FUNCTION_BLOCK FB_SortingModule EXTENDS FB_Module
// Module to select via sensor, cylinder and axis
VAR_INPUT
		(* Variables to enable / disable diagnosis and temperature mode *)
	bCylinderDiag				: BOOL;
	bCylinderTemp				: BOOL;
	bCylinderRecord				: BOOL;
		(* Buttons *)
	bButtonCylToWorkIn			: BOOL;
	bButtonCylToBaseIn			: BOOL;
		(* Timer values *)
	tTimeOutCylinder			: TIME;
	tRecordIntervall			: TIME;
	tSensorDelay				: TIME;
	tMoveAxis					: TIME;					// Time to move axis
END_VAR
VAR_OUTPUT
	bToWork						: BOOL;
	bAtBase						: BOOL;
	bAtWork						: BOOL;
	bCylError					: BOOL;
	sCylErrorMsg				: STRING;
	aTemps						: ARRAY[1..100] OF LREAL;
	bSelected					: BOOL;
	bButtonCylToWorkOut			: BOOL;
	bButtonCylToBaseOut			: BOOL;
END_VAR
VAR
(* ================= Function block and interface instances ===================== *)
	
	fbSensorDelay				: FB_SignalHandlingDelay;
		(* Instances of cylinder function blocks *)
	fbCylinder					: FB_Cylinder;					// Without diagnosis and temperature mode
	fbCylinderDiag				: FB_CylinderDiag;				// With diagnosis of states
	fbCylinderTemp				: FB_CylinderTemp;				// With temperature mode
	fbCylinderTempDiag			: FB_CylinderTempDiag;			// With diagnosis of temperature
	fbCylinderTempRecord		: FB_CylinderTempRecord;		// With record of temperatures
		(* Interface instance of ICylinder for cylinder *)
	iCyl						: ICylinder;
	
		(***** Manual cylinder control *****)
	fbButtonCylToWork			: FB_SignalHandlingIntern;		// To move manually cylinder to work position
	fbButtonCylToBase			: FB_SignalHandlingIntern;		// To move manually cylinder to base position

(* ========================== COMMON VARIABLES =============================== *)
	fbTimerAxis					: TON;							// Timer to move axis in (SEMI-) AUTOMATIC mode	
	fbTriggerCylAtWork			: R_TRIG;						// To diagnose rising edge of being in work position
	eStateAuto					: E_StateSortingAuto;
END_VAR

// =========================================================
;
// =========================================================

METHOD PROTECTED M_ResetState
VAR_INPUT
END_VAR
// =========================================================

eStateAuto := eSortingAuto_DetectBox;

// =========================================================
END_METHOD

METHOD PUBLIC M_SetOutput
VAR_INPUT
END_VAR
// =========================================================
		// Calling method M_SetOutput of base class FB_Module via 'SUPER^.'
		
SUPER^.M_SetOutput();

// =========================================================
		// Sensor
		
fbSensorDelay.M_SetOutput();

// =========================================================
		// Cylinder buttons
		
fbButtonCylToWork.M_SetOutput();
fbButtonCylToBase.M_SetOutput();

// =========================================================
		// Output variables for cylinder
		
bToWork := iCyl.P_ToWork;			// Assigning global output variable to property of selected FB
									// Accessing property of selected FB via interface instance
bAtBase := iCyl.P_AtBasePos;
bAtWork := iCyl.P_AtWorkPos;

// =========================================================
		// Buttons
		
fbButtonCylToWork.bInput 	:= bButtonCylToWorkIn;
fbButtonCylToBase.bInput	:= bButtonCylToBaseIn;
bButtonCylToWorkOut 		:= fbButtonCylToWork.bOut;
bButtonCylToBaseOut 		:= fbButtonCylToBase.bOut;

// =========================================================
END_METHOD

METHOD PUBLIC M_Automatic
VAR_INPUT
END_VAR
// =========================================================
		// Selecting boxes via cylinder and axis

fbTimerAxis( PT := tMoveAxis );
fbTriggerCylAtWork( CLK := iCyl.P_AtWorkPos );			(***** Accessing property of FB via interface *****)

IF fbTriggerCylAtWork.Q THEN
	fbTimerAxis( IN := TRUE );
END_IF

IF bSelected THEN
	bSelected := FALSE;
END_IF

IF fbTimerAxis.Q THEN
	fbTimerAxis( IN := FALSE );
	
	bSelected 	:= TRUE;
	bHalt 		:= TRUE;
	
	M_Stop();
	
ELSIF fbTimerAxis.IN AND NOT bHalt THEN
	fbAxis.M_MoveFw();
END_IF

IF NOT bHaltDone THEN
	
	IF bHalt THEN
		M_Stop();
	END_IF
ELSE
	bHalt := FALSE;
	M_Stop();
END_IF

// =========================================================

CASE eStateAuto OF
	// =========================================================
	// Detecting a box
	eSortingAuto_DetectBox:	
	
			iCyl.M_MoveToBase();						(***** Calling method of FB via interface *****)
			
			IF fbSensorDelay.bOut THEN
				eStateAuto := eSortingAuto_CylToWork;
			END_IF
		
	// =========================================================
	// Moving cylinder to work position
	eSortingAuto_CylToWork:
	
			iCyl.M_MoveToWork();						(***** Calling method of FB via interface *****)
			
			IF iCyl.P_AtWorkPos THEN					(***** Accessing property of FB via interface *****)
				eStateAuto := eSortingAuto_CylToBase;
			END_IF
	
	// =========================================================
	// Moving cylinder back to base position
	eSortingAuto_CylToBase:
	
			iCyl.M_MoveToBase();						(***** Calling method of FB via interface *****)	
			
			IF iCyl.P_AtBasePos THEN					(***** Accessing property of FB via interface *****)
				eStateAuto := eSortingAuto_DetectBox;
			END_IF
END_CASE

// =========================================================
END_METHOD

METHOD PUBLIC M_Manual
VAR_INPUT
END_VAR
// =========================================================
		// Calling method M_Manual of base class FB_Module via 'SUPER^.'
		
SUPER^.M_Manual();

// =========================================================
	// Manual cylinder control
	
IF fbButtonCylToWork.bOut THEN
	iCyl.M_MoveToWork();				(**** Calling method of FB via interface instance ****)
	
ELSIF fbButtonCylToBase.bOut THEN
	iCyl.M_MoveToBase();				(**** Calling method of FB via interface instance ****)
END_IF

// =========================================================
END_METHOD

METHOD PUBLIC M_CylinderOptions
VAR_INPUT
END_VAR
// =========================================================
			// Selecting cylinder

// Checking variables to enable / disable diagnosis and temperature mode
IF bCylinderDiag THEN
	
	IF bCylinderTemp THEN
		
	(* ============== FB with diagnosis and temperature mode ============== *)
		bCylError 		:= fbCylinderTempDiag.bError;				// Assigning global output variable to output variable of selected FB
		sCylErrorMsg 	:= fbCylinderTempDiag.sErrorMsg;
		iCyl 			:= fbCylinderTempDiag;						// Assigning desired FB instance to interface instance
	
	ELSE
	
	(* ============== FB with diagnosis and without temperature mode ============== *)
		fbCylinderDiag.tTimeOut 	:= tTimeOutCylinder;			// Setting special data for selected FB
		bCylError 					:= fbCylinderDiag.bError;		// Assigning global output variable to output variable of selected FB
		sCylErrorMsg 				:= fbCylinderDiag.sErrorMsg;
		iCyl 						:= fbCylinderDiag;				// Assigning desired FB instance to interface instance
	END_IF
	
ELSE
	bCylError 		:= FALSE;
	sCylErrorMsg 	:= '';
	
	IF bCylinderTemp THEN
		
		IF bCylinderRecord THEN
			fbCylinderTempRecord.tIntervalTime	:= tRecordIntervall;	// Time of record interval
			fbCylinderTempRecord.bRecordStart 	:= bComprAirEnabled;	// Recording if compressed air is set
			
			fbCylinderTempRecord.M_Record();							// Calling method of function block FB_CylinderTempRecord
			
			aTemps	:= fbCylinderTempRecord.aTemps;					// Saving output variable
			iCyl 	:= fbCylinderTempRecord;
		ELSE
			(* ============== FB without diagnosis and with temperature mode ============== *)
			iCyl := fbCylinderTemp; 						// Assigning desired FB instance to interface instance
		END_IF
		
	ELSE
	(* ============== FB without diagnosis and temperature mode ============== *)
		iCyl := fbCylinder;							// Assigning desired FB instance to interface instance						
	END_IF	
END_IF
									
// =========================================================
END_METHOD

METHOD PUBLIC M_Enable
VAR_INPUT
END_VAR
// =========================================================
		// Calling method M_Enable of base class FB_Module via 'SUPER^.'
		
SUPER^.M_Enable();

// =========================================================
		// Sensor control
		
fbSensorDelay.bEnable := bSensorEnable;

// =========================================================
		// Cylinder control
		
fbButtonCylToWork.bEnable 	:= bManualCylinderEnable
								AND NOT iCyl.P_AtWorkPos;		(*** Accessing property of FB via interface instance ***)
								
fbButtonCylToBase.bInput 	:= NOT fbButtonCylToWork.bInput;

fbButtonCylToBase.bEnable 	:= bManualCylinderEnable
								AND NOT iCyl.P_AtBasePos;		(*** Accessing property of FB via interface instance ***)

// =========================================================
END_METHOD

METHOD PUBLIC M_Maintenance
VAR_INPUT
END_VAR
// =========================================================
		// Calling own method M_Manual of this class FB_SortingModule via 'THIS^.'
		
THIS^.M_Manual();

// =========================================================
END_METHOD

METHOD PUBLIC M_Reset
VAR_INPUT
END_VAR
// =========================================================
		// Resetting cylinder and axis
		
fbTriggerResetStart( CLK := bReset );

IF fbTriggerResetStart.Q THEN
	bSelected := FALSE;
	
	fbTimerAxis( IN := FALSE );
	
	iCyl.M_Reset();						(**** Calling method of FB via interface ****)
END_IF

// =========================================================
		// Calling method of base class
		
SUPER^.M_Reset();						// Calling action M_Reset of base class FB_Module via 'SUPER^.'

// =========================================================
END_METHOD

METHOD PUBLIC M_Semiautomatic
VAR_INPUT
END_VAR
// =========================================================
		// Calling own method M_Automatic of this class FB_SortingModule via 'THIS^.'
		
THIS^.M_Automatic();				

// =========================================================
END_METHOD

METHOD PUBLIC M_Starting
VAR_INPUT
END_VAR
// =========================================================
		// Setting time to delay sensor
		
fbSensorDelay.tDelay := tSensorDelay;

// =========================================================
		// Calling method M_Starting of base class FB_Module via 'SUPER^.'
		
SUPER^.M_Starting();

// =========================================================
END_METHOD

END_FUNCTION_BLOCK
